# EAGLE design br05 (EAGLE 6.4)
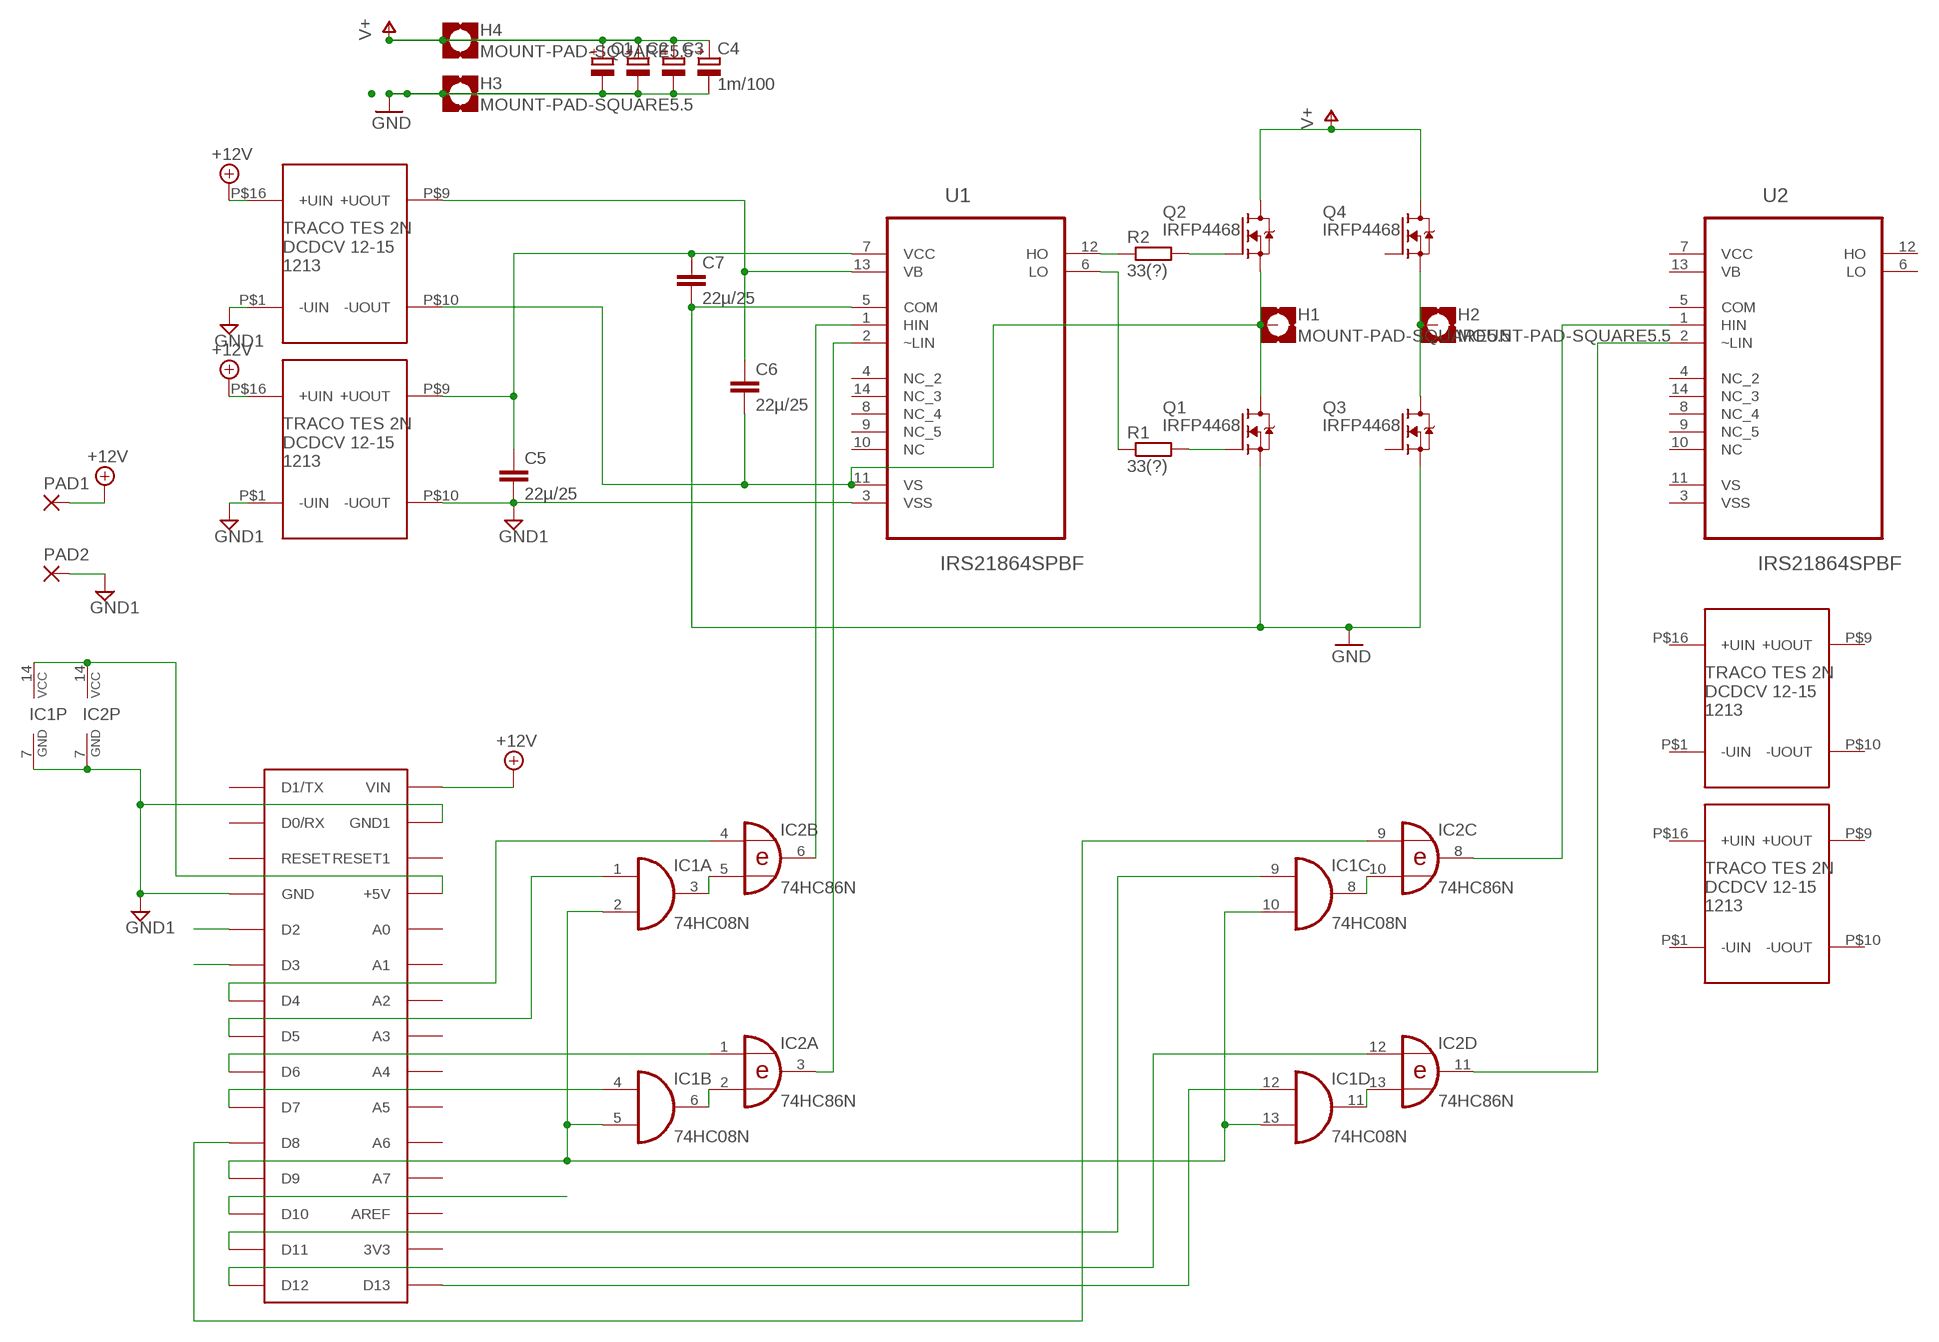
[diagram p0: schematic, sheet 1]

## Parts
C1  CPOL-EUE10-25  [EB25D]
C2  CPOL-EUE10-25  [EB25D]
C3  CPOL-EUE10-25  [EB25D]
C4  1m/100  CPOL-EUE10-25  [EB25D]
C5  22µ/25  C-EUC1210  [C1210]
C6  22µ/25  C-EUC1210  [C1210]
C7  22µ/25  C-EUC1210  [C1210]
H1  MOUNT-PAD-SQUARE5.5  [5,5-PAD-SQUARE]
H2  MOUNT-PAD-SQUARE5.5  [5,5-PAD-SQUARE]
H3  MOUNT-PAD-SQUARE5.5  [5,5-PAD-SQUARE]
H4  MOUNT-PAD-SQUARE5.5  [5,5-PAD-SQUARE]
IC1  74HC08N  [DIL14]
IC2  74HC86N  [DIL14]
PAD1  2,54/1,1  [2,54/1,1]
PAD2  2,54/1,1  [2,54/1,1]
Q1  IRFP4468  [TO247]
Q2  IRFP4468  [TO247]
Q3  IRFP4468  [TO247]
Q4  IRFP4468  [TO247]
R1  33(?)  R-EU_R2012  [R2012]
R2  33(?)  R-EU_R2012  [R2012]
U1  IRS21864SPBF  [SOIC127P600X175-14N]
U2  IRS21864SPBF  [SOIC127P600X175-14N]
U$1  TES21215TES_2N_1213  [TES_2]
U$2  TES21215TES_2N_1213  [TES_2]
U$3  TES21215TES_2N_1213  [TES_2]
U$4  ARDUINONANO  [PDIP-32]
U$11  TES21215TES_2N_1213  [TES_2]

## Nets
+12V: PAD1.1(P) U$1.P$16(+UIN) U$4.VIN U$11.P$16(+UIN)
GND: C1.- C2.- C3.- C4.- C7.2 H3.B5,5(MOUNT) Q1.S Q3.S U1.5(COM)
GND1: C5.2 IC1.7(P:GND) IC2.7(P:GND) PAD2.1(P) U1.3(VSS) U$1.P$1(-UIN) U$1.P$10(-UOUT) U$4.GND U$4.GND1 U$11.P$1(-UIN)
HO1: R2.1 U1.12(HO)
INT0: U$4.D2
INT1: U$4.D3
LO1: R1.1 U1.6(LO)
M1: C6.2 H1.B5,5(MOUNT) Q1.D Q2.S U1.11(VS) U$11.P$10(-UOUT)
M2: H2.B5,5(MOUNT) Q3.D Q4.S
N$2: Q2.G R2.2
N$3: Q1.G R1.2
N$8: C6.1 U1.13(VB) U$11.P$9(+UOUT)
N$9: IC2.6(B:O) U1.1(HIN)
N$10: IC2.3(A:O) U1.2(~LIN)
N$11: C5.1 C7.1 U1.7(VCC) U$1.P$9(+UOUT)
N$16: IC2.4(B:I0) U$4.D4
N$17: IC1.1(A:I0) U$4.D5
N$18: IC2.1(A:I0) U$4.D6
N$19: IC1.4(B:I0) U$4.D7
N$20: IC1.12(D:I0) U$4.D13
N$21: IC2.12(D:I0) U$4.D12
N$22: IC1.3(A:O) IC2.5(B:I1)
N$23: IC1.6(B:O) IC2.2(A:I1)
N$24: IC1.11(D:O) IC2.13(D:I1)
N$25: IC1.8(C:O) IC2.10(C:I1)
N$26: IC1.9(C:I0) U$4.D11
N$27: IC2.9(C:I0) U$4.D8
N$28: IC2.8(C:O) U2.1(HIN)
N$29: IC2.11(D:O) U2.2(~LIN)
N$30: IC1.14(P:VCC) IC2.14(P:VCC) U$4.+5V
PWM1: IC1.2(A:I1) IC1.5(B:I1) IC1.10(C:I1) IC1.13(D:I1) U$4.D9
PWM2_STROMMESS: U$4.D10
V+: C1.+ C2.+ C3.+ C4.+ H4.B5,5(MOUNT) Q2.D Q4.D
Unconnected: Q3.G Q4.G U1.4(NC_2) U1.8(NC_4) U1.9(NC_5) U1.10(NC) U1.14(NC_3) U2.4(NC_2) U2.5(COM) U2.6(LO) U2.8(NC_4) U2.9(NC_5) U2.10(NC) U2.12(HO) U2.13(VB) U2.14(NC_3) U$2.P$1(-UIN) U$2.P$9(+UOUT) U$2.P$10(-UOUT) U$2.P$16(+UIN) U$3.P$1(-UIN) U$3.P$9(+UOUT) U$3.P$10(-UOUT) U$3.P$16(+UIN) U$4.3V3 U$4.A0 U$4.A1 U$4.A2 U$4.A3 U$4.A4 U$4.A5 U$4.A6 U$4.A7 U$4.AREF U$4.D0/RX U$4.D1/TX U$4.RESET U$4.RESET1

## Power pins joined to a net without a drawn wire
VCC: U2.7(VCC)
VS: U2.11(VS)
VSS: U2.3(VSS)

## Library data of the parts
C1-C4 = rcl:CPOL-EU: POLARIZED CAPACITOR, European symbol
C5-C7 = resistor:C-EU: CAPACITOR, European symbol
H1-H4 = holes:MOUNT-PAD-SQUARE: MOUNTING PAD, square
IC1 = 74xx-eu:74*08: Quad 2-input AND gate
IC2 = 74xx-eu:74*86: Quad 2-input EXCLUSIVE-OR (XOR) gate
PAD1 PAD2 = wirepad:2,54/1,1: THROUGH-HOLE PAD
Q1-Q4 = div-wo:IRFP4468
R1 R2 = resistor:R-EU_: RESISTOR, European symbol
U1 U2 = International_Rectifier_By_element14_Batch_1:IRS21864SPBF: HIGH AND LOW SIDE DRIVER; MPN: IRS21864SPBF; OC_FARNELL: 1688539; OC_NEWARK: 21M6614; PACKAGE: SOIC-14; SUPPLIER: International Rectifier
U$1-U$3 U$11 = div-wo:TES21215: Traco Power DCDC Konverter TES 2N Serie, 2Watt
U$4 = jet-lib:ARDUINONANO

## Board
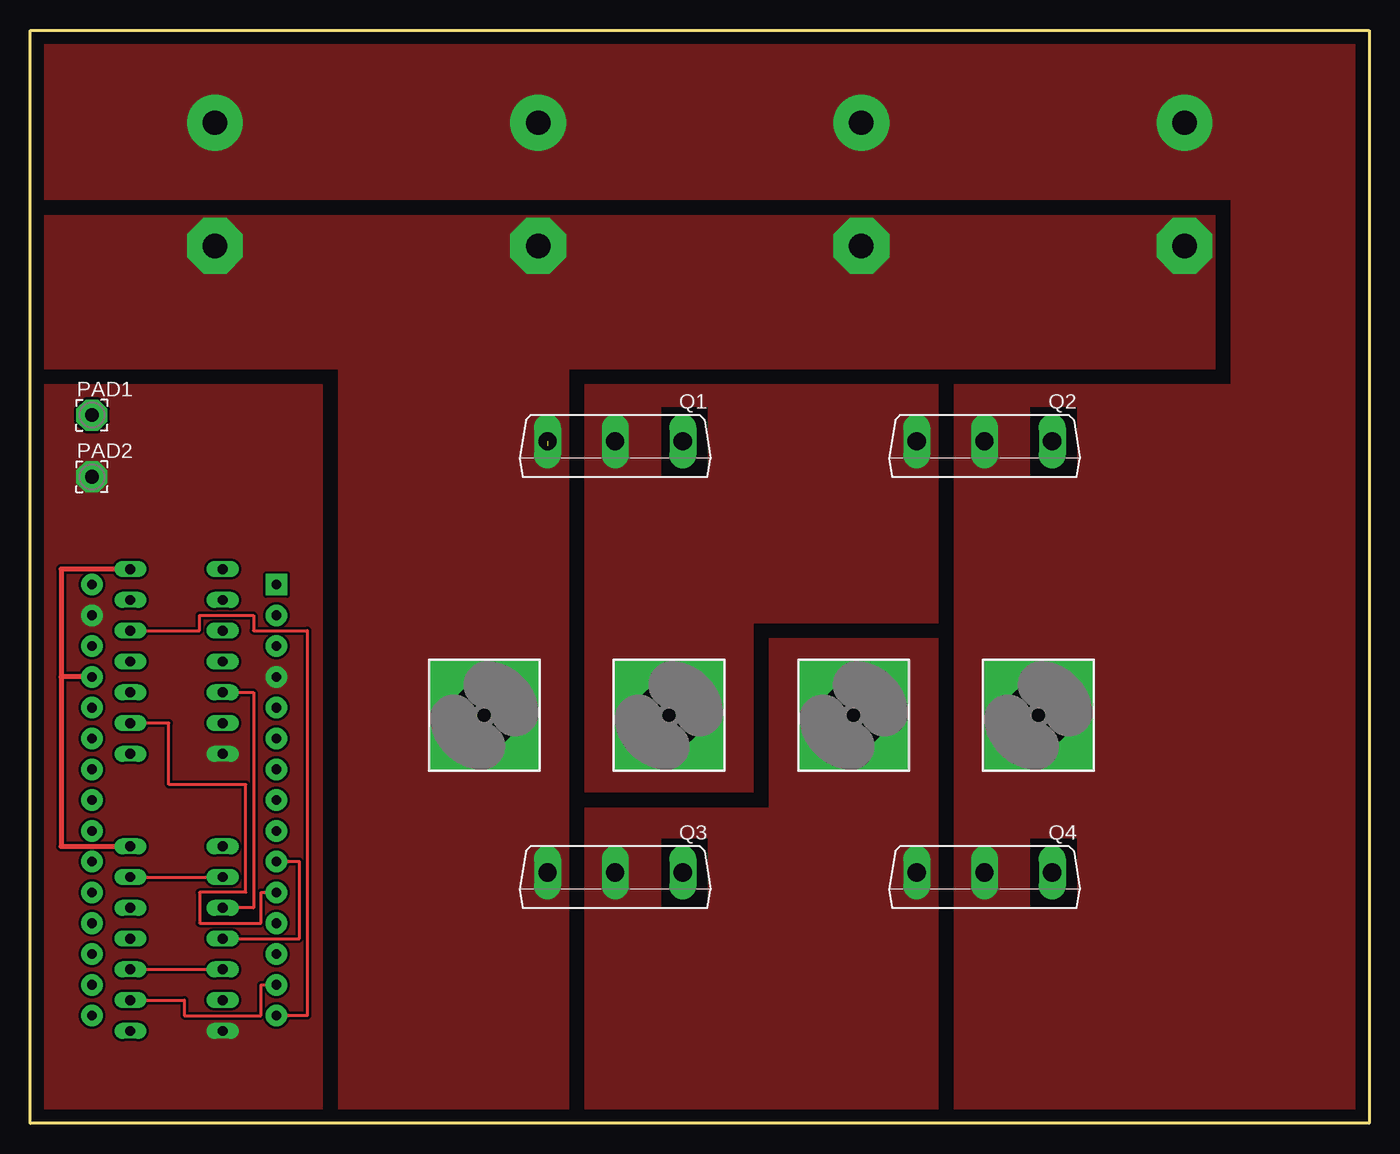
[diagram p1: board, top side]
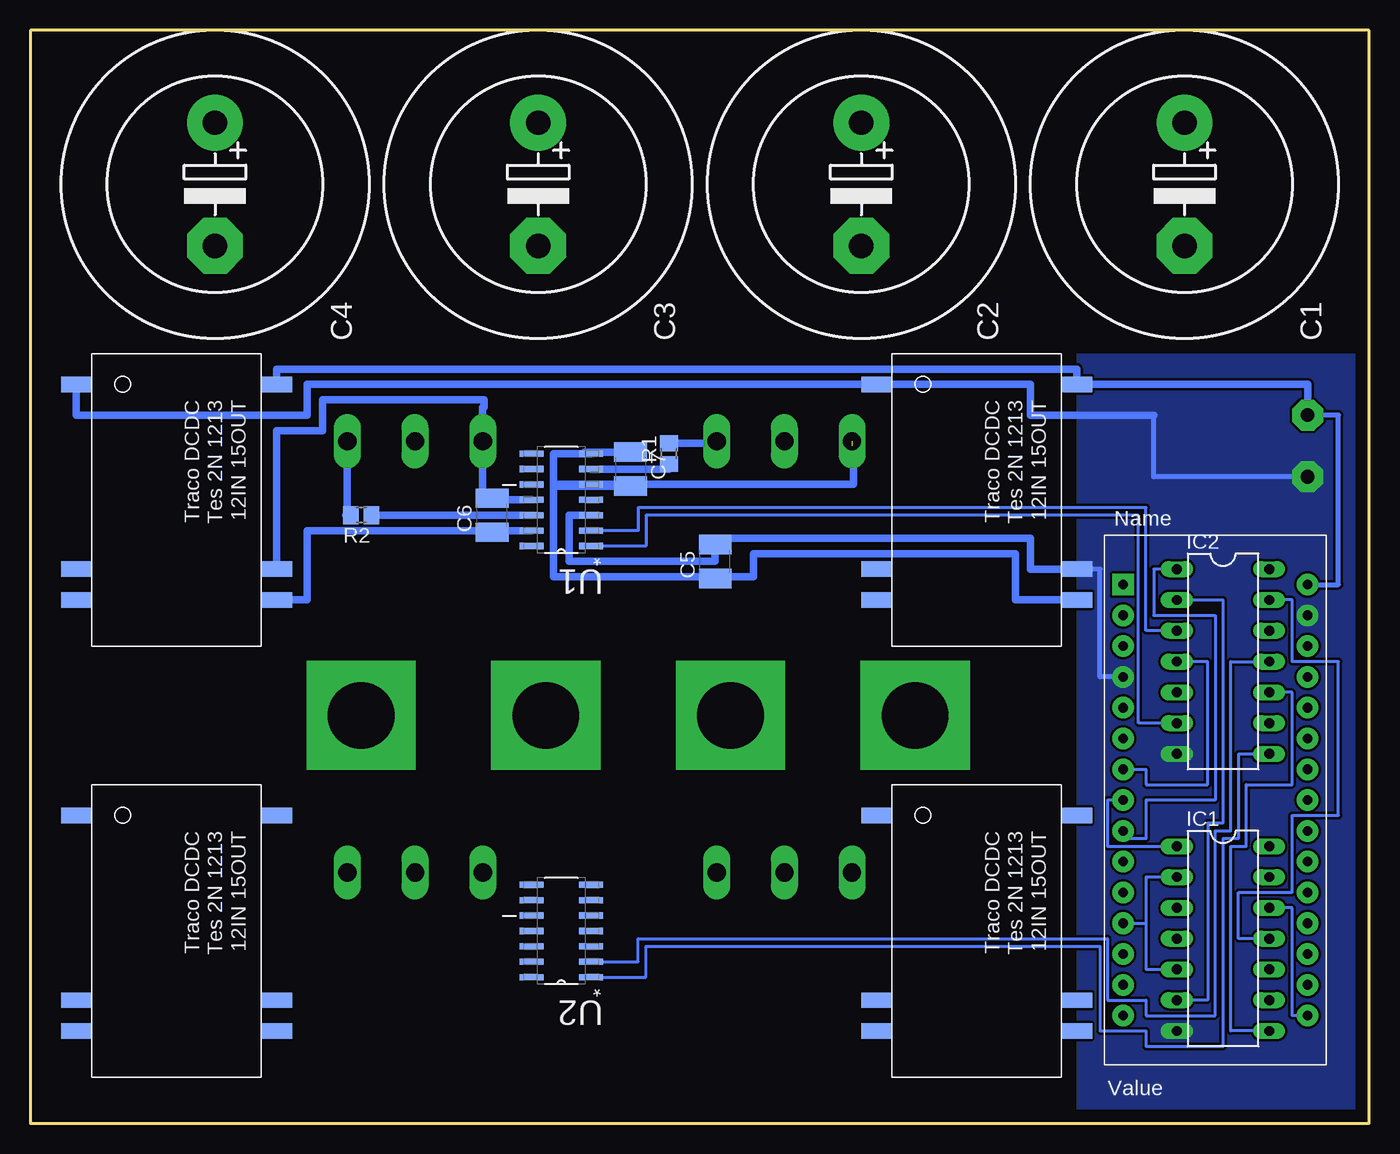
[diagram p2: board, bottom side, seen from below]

Size 110.49 x 90.17 mm. Coordinates in mm from the lower left corner, seen from the top.
Outline: 0,90.17 110.49,90.17 110.49,0 0,0 0,90.17
Copper layers (1*16): Top 0.035mm / dielectric 1.5mm / Bottom 0.035mm
Design rules "default": minimum track width 10mil, minimum drill 24mil, track to track 8mil, track to pad 8mil, pad to pad 8mil, via to via 8mil, smd to smd 8mil, copper to edge 40mil, drill to drill 8mil, minimum pad ring 10mil, minimum via ring 8mil, stop-mask expansion 4mil, vias tented up to drill 0mil, thermal gap 10mil

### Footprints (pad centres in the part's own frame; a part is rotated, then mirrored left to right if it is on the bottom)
EB25D = drill 2.007 pad 4.597: + -5.08,0 | drill 2.007 pad 4.597 octagon: - 5.08,0
C1210 = smd 1.6 x 2.7: 1 -1.4,0; 2 1.4,0
5,5-PAD-SQUARE = drill 5.5 pad 9 square: B5,5 0,0
DIL14 = drill 0.813 long: 1 -7.62,-3.81; 2 -5.08,-3.81; 3 -2.54,-3.81; 4 0,-3.81; 5 2.54,-3.81; 6 5.08,-3.81; 7 7.62,-3.81; 8 7.62,3.81; 9 5.08,3.81; 10 2.54,3.81; 11 0,3.81; 12 -2.54,3.81; 13 -5.08,3.81; 14 -7.62,3.81
2,54/1,1 = drill 1.118 pad 2.54 octagon: 1 0,0
TO247 = drill 1.499 long: D 0,-0.381; G -5.588,-0.381; S 5.588,-0.381
R2012 = smd 1.3 x 1.5: 1 -0.85,0; 2 0.85,0
SOIC127P600X175-14N = smd 1.981 x 0.508: 1 -2.464,3.81; 2 -2.464,2.54; 3 -2.464,1.27; 4 -2.464,0; 5 -2.464,-1.27; 6 -2.464,-2.54; 7 -2.464,-3.81; 8 2.464,-3.81; 9 2.464,-2.54; 10 2.464,-1.27; 11 2.464,0; 12 2.464,1.27; 13 2.464,2.54; 14 2.464,3.81
TES_2 = smd 1.27 x 2.54: P$1 2.54,-15.24; P$2 2.54,1.27; P$7 17.78,-15.24; P$8 20.32,-15.24; P$9 20.32,1.27; P$10 17.78,1.27; P$16 2.54,1.27
PDIP-32 = drill 0.8 pad 1.778: 3V3 15.24,-35.56; +5V 15.24,-10.16; A0 15.24,-12.7; A1 15.24,-15.24; A2 15.24,-17.78; A3 15.24,-20.32; A4 15.24,-22.86; A5 15.24,-25.4; A6 15.24,-27.94; A7 15.24,-30.48; AREF 15.24,-33.02; D0/RX 0,-5.08; D2 0,-12.7; D3 0,-15.24; D4 0,-17.78; D5 0,-20.32; D6 0,-22.86; D7 0,-25.4; D8 0,-27.94; D9 0,-30.48; D10 0,-33.02; D11 0,-35.56; D12 0,-38.1; D13 15.24,-38.1; GND 0,-10.16; GND1 15.24,-5.08; RESET 0,-7.62; RESET1 15.24,-7.62; VIN 15.24,-2.54 | drill 0.8 pad 1.778 square: D1/TX 0,-2.54

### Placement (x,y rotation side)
C1  15.24,77.47 270 bottom
C2  41.91,77.47 270 bottom
C3  68.58,77.47 270 bottom
C4  95.25,77.47 270 bottom
C5  53.98,46.36 90 bottom
C6  72.39,50.17 90 bottom
C7  60.96,53.98 270 bottom
H1  52.7,33.66 0 top
H2  67.95,33.66 0 top
H3  37.46,33.66 0 top
H4  83.19,33.66 0 top
IC1  12.07,15.24 270 bottom
IC2  12.07,38.1 270 bottom
PAD1  5.08,58.42 0 top
PAD2  5.08,53.34 0 top
Q1  48.26,55.88 180 top
Q2  78.74,55.88 180 top
Q3  48.26,20.32 180 top
Q4  78.74,20.32 180 top
R1  57.78,55.25 90 bottom
R2  83.19,50.17 180 bottom
U1  66.67,51.44 180 bottom
U2  66.67,15.88 180 bottom
U$1  25.4,63.5 270 bottom
U$2  91.44,27.94 270 bottom
U$3  25.4,27.94 270 bottom
U$4  20.32,46.99 0 bottom
U$11  91.44,63.5 270 bottom

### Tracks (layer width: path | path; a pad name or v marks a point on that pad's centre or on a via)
+12V
  Bottom 0.406: U$4.VIN 2.54,44.45 2.54,58.42 PAD1.1
  Bottom 0.61: U$11.P$16 90.17,62.23 24.13,62.23 U$1.P$16 5.08,60.96 PAD1.1
GND  (1 unrouted)
  Bottom 0.61: 42.67,55.88 42.55,55.88 42.55,52.71 U1.5 67.31,52.71 67.31,52.58 C7.2
  pour Top (isolate 0.61, no thermals): 44.45,62.23 97.79,62.23 97.79,74.93 0,74.93 0,62.23 25.4,62.23 25.4,0 44.45,0
GND1
  Bottom 0.406: PAD2.1 17.78,53.34 17.78,58.42 | U$4.GND 22.23,36.83 22.23,45.72 U$1.P$10
  Bottom 0.61: U$1.P$10 27.94,45.72 27.94,48.26 53.98,48.26 C5.2 53.98,46.36 66.04,46.36 66.04,50.17 U1.3 | 17.78,58.42 27.94,58.42 27.94,60.96 U$1.P$1 87.63,60.96 87.63,58.42 106.68,58.42 U$11.P$1
  pour Top (no thermals): 0,0 24.13,0 24.13,60.96 0,60.96
  pour Bottom (no thermals): 0,63.5 24.13,63.5 24.13,0 0,0
HO1
  Bottom 0.61: U1.12 R2.1
LO1
  Bottom 0.61: U1.6 57.78,53.98 R1.1
M1
  Bottom 0.61: U1.11 72.39,51.44 | C6.2 72.39,51.44 | 72.39,51.44 73.15,51.44 Q2.S 73.15,59.05 73.02,59.05 73.02,59.69 86.36,59.69 86.36,57.15 90.17,57.15 U$11.P$10
  pour Top (no thermals): 45.72,60.96 74.93,60.96 74.93,41.28 59.69,41.28 59.69,27.3 45.72,27.3
M2
  pour Top (no thermals): 45.72,26.04 60.96,26.04 60.96,40.01 74.93,40.01 74.93,0 45.72,0
N$1
  cutout Top: 52.07,59.05 55.88,59.05 55.88,53.34 52.07,53.34
  cutout Top: 82.55,59.05 86.36,59.05 86.36,53.34 82.55,53.34
  cutout Top: 52.07,23.5 55.88,23.5 55.88,17.78 52.07,17.78
  cutout Top: 86.36,23.5 82.55,23.5 82.55,17.78 86.36,17.78
N$2
  Bottom 0.61: R2.2 84.33,50.17 | 84.45,50.17 84.33,50.17 | 84.33,50.17 Q2.G
N$3
  Bottom 0.61: R1.2 53.85,56.1 Q1.G
N$8
  Bottom 0.61: U1.13 73.02,48.9 C6.1 72.39,48.9 87.63,48.9 87.63,43.18 U$11.P$9
N$9
  Bottom 0.254: IC2.6 19.05,33.02 19.05,50.17 59.69,50.17 59.69,47.62 U1.1
N$10
  Bottom 0.254: IC2.3 18.41,40.64 18.41,50.8 60.32,50.8 60.32,48.9 U1.2
N$11
  Bottom 0.61: U1.7 64.77,55.25 | 64.77,55.25 67.31,55.25 67.31,45.09 53.34,45.09 | 53.34,45.09 C5.1 | U$1.P$9 29.21,43.18 29.21,46.99 50.8,46.99 50.8,45.09 53.34,45.09 | C7.1 64.77,55.38 64.77,55.25
N$16
  Bottom 0.254: U$4.D4 18.41,29.21 18.41,27.94 13.34,27.94 13.34,38.1 IC2.4
N$17
  Bottom 0.254: U$4.D5 21.59,26.67 21.59,22.86 IC1.1
N$18
  Bottom 0.254: IC2.1 17.78,45.72 17.78,41.91 12.7,41.91 12.7,26.67 18.41,26.67 18.41,23.5 20.32,23.5 U$4.D6
N$19
  Top 0.254: IC1.4 22.23,15.24 22.23,21.59 U$4.D7
N$20
  Bottom 0.254: U$4.D13 6.35,8.89 6.35,17.78 IC1.12
N$21
  Top 0.254: U$4.D12 22.86,8.89 22.86,40.64 18.41,40.64 18.41,41.91 13.97,41.91 13.97,40.64 IC2.12
N$22
  Top 0.254: IC2.5 18.41,35.56 18.41,17.78 IC1.3
N$23
  Bottom 0.254: IC2.2 12.07,43.18 12.07,24.77 13.34,24.77 13.34,10.16 IC1.6
N$24
  Bottom 0.254: IC1.11 10.79,15.24 10.79,19.05 6.35,19.05 6.35,25.4 2.54,25.4 2.54,38.1 6.35,38.1 6.35,43.18 IC2.13
N$25
  Bottom 0.254: IC1.8 11.43,7.62 11.43,22.86 10.16,22.86 10.16,27.94 6.35,27.94 6.35,35.56 IC2.10
N$26
  Top 0.254: IC1.9 12.7,10.16 12.7,8.89 19.05,8.89 19.05,11.43 U$4.D11
N$27
  Top 0.254: IC2.9 11.43,33.02 11.43,27.94 17.78,27.94 17.78,19.05 13.97,19.05 13.97,16.51 19.05,16.51 19.05,19.05 U$4.D8
N$28
  Bottom 0.254: U2.1 59.69,12.06 59.69,14.61 22.23,14.61 22.23,7.62 18.41,7.62 18.41,6.35 12.07,6.35 12.07,23.5 10.79,23.5 10.79,30.48 IC2.8
N$29
  Bottom 0.254: U2.2 60.32,13.33 60.32,15.24 21.59,15.24 21.59,10.16 18.41,10.16 18.41,8.89 12.7,8.89 12.7,24.13 11.43,24.13 11.43,38.1 IC2.11
N$30
  Top 0.406: IC2.14 2.54,45.72 2.54,36.83 | U$4.+5V 2.54,36.83 | 2.54,36.83 2.54,22.86 IC1.14
PWM1
  Top 0.254: IC1.10 IC1.5 | IC1.13 IC1.2
  Bottom 0.254: IC1.2 18.41,20.32 18.41,16.51 | U$4.D9 18.41,16.51 | 18.41,16.51 18.41,12.7 IC1.5
V+
  pour Top (no thermals): 76.2,60.96 99.06,60.96 99.06,76.2 0,76.2 0,90.17 110.49,90.17 110.49,0 76.2,0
